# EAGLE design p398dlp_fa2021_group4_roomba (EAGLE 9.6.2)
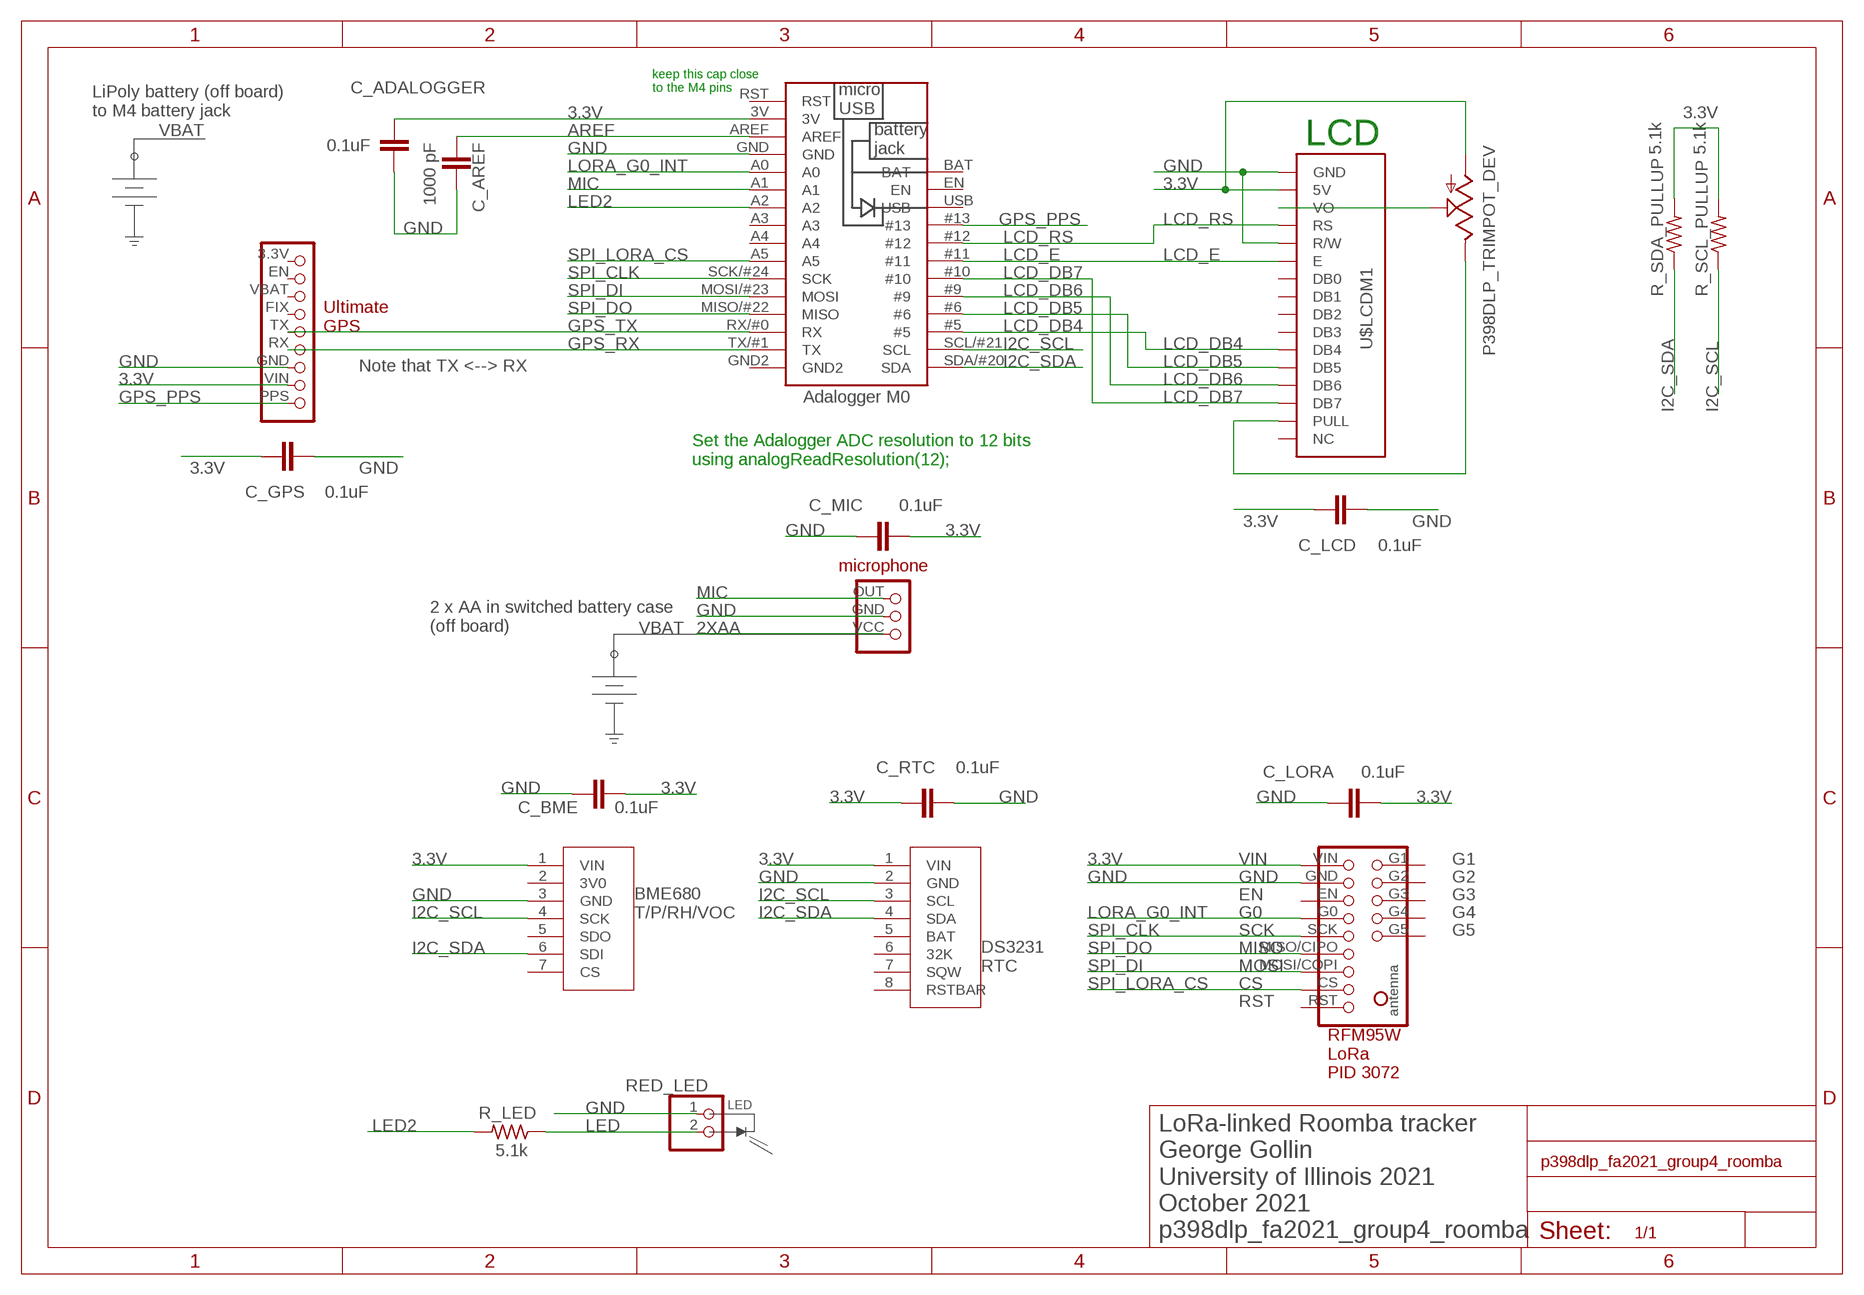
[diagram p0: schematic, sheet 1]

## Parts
BME  P398DLP_BME680_DEV  [P398DLP_BME680_PKG]
C_ADALOGGER  0.1uF  C5/3.5  [C5B3.5]
C_AREF  1000 pF  C5/3.5  [C5B3.5]
C_BME  0.1uF  C5/3.5  [C5B3.5]
C_GPS  0.1uF  C5/3.5  [C5B3.5]
C_LCD  0.1uF  C5/3.5  [C5B3.5]
C_LORA  0.1uF  C5/3.5  [C5B3.5]
C_MIC  0.1uF  C5/3.5  [C5B3.5]
C_RTC  0.1uF  C5/3.5  [C5B3.5]
DS3231  P398DLP_DS3231_DEV  [P398DLP_DS3231_PKG]
R_LED  5.1k  R-US_0207/7  [0207/7]
R_SCL_PULLUP  5.1k  R-US_0207/7  [0207/7]
R_SDA_PULLUP  5.1k  R-US_0207/7  [0207/7]
RED_LED  LED  PINHD-1X2  [1X02]
RFM95W  P398DLP_LORA_BREAKOUT_DEV  [P398DLP_LORA_BREAKOUT_PKG]
TRIMPOTADL1  P398DLP_TRIMPOT_DEV  [P398DLP_TRIMPOT_PKG]
U$2  P398DLP_ADALOGGER_MO_DEV  [P398DLP_ADALOGGER_M0_PKG]
U$7  P398DLP_MICROPHONE_DEV  [P398DLP_MICROPHONE_PKG]
U$16  P398DLP_ULTIMATE_GPS_DEV  [P398DLP_ULTIMATE_GPS_PKG]
U$LCDM1  P398DLP_LCD_16X2_DEV  [P398DLP_LCD_16X2_PKG]

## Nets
2XAA [power]: U$7.VCC
3.3V [power]: BME.1(VIN) C_ADALOGGER.1 C_BME.2 C_GPS.2 C_LCD.2 C_LORA.2 C_MIC.2 C_RTC.2 DS3231.1(VIN) R_SCL_PULLUP.2 R_SDA_PULLUP.2 RFM95W.VIN TRIMPOTADL1.BOTTOM U$2.3V U$16.VIN U$LCDM1.5V
AREF: C_AREF.1 U$2.AREF
GND [power]: BME.3(GND) C_ADALOGGER.2 C_AREF.2 C_BME.1 C_GPS.1 C_LCD.1 C_LORA.1 C_MIC.1 C_RTC.1 DS3231.2(GND) RED_LED.1 RFM95W.GND U$2.GND U$7.GND U$16.GND U$LCDM1.GND U$LCDM1.R/W
GPS_PPS: U$2.#13 U$16.PPS
GPS_RX: U$2.TX/#1(TX) U$16.RX
GPS_TX: U$2.RX/#0(RX) U$16.TX
I2C_SCL: BME.4(SCK) DS3231.3(SCL) R_SCL_PULLUP.1 U$2.SCL/#21(SCL)
I2C_SDA: BME.6(SDI) DS3231.4(SDA) R_SDA_PULLUP.1 U$2.SDA/#20(SDA)
LCD_DB4: U$2.#5 U$LCDM1.DB4
LCD_DB5: U$2.#6 U$LCDM1.DB5
LCD_DB6: U$2.#9 U$LCDM1.DB6
LCD_DB7: U$2.#10 U$LCDM1.DB7
LCD_E: U$2.#11 U$LCDM1.E
LCD_RS: U$2.#12 U$LCDM1.RS
LED2: R_LED.2 U$2.A2
LORA_G0_INT: RFM95W.G0 U$2.A0
MIC: U$2.A1 U$7.OUT
N$1: TRIMPOTADL1.TAP U$LCDM1.VO
N$4: TRIMPOTADL1.TOP U$LCDM1.PULL
N$34: R_LED.1 RED_LED.2
SPI_CLK: RFM95W.SCK U$2.SCK/#24(SCK)
SPI_DI: RFM95W.MOSI/COPI(MOSI) U$2.MOSI/#23(MOSI)
SPI_DO: RFM95W.MISO/CIPO(MISO) U$2.MISO/#22(MISO)
SPI_LORA_CS: RFM95W.CS U$2.A5
Unconnected: BME.2(3V0) BME.5(SDO) BME.7(CS) DS3231.5(BAT) DS3231.6(32K) DS3231.7(SQW) DS3231.8(RSTBAR) RFM95W.EN RFM95W.G1 RFM95W.G2 RFM95W.G3 RFM95W.G4 RFM95W.G5 RFM95W.RST U$2.A3 U$2.A4 U$2.BAT U$2.EN U$2.GND2 U$2.RST U$2.USB U$16.3.3V U$16.EN U$16.FIX U$16.VBAT U$LCDM1.DB0 U$LCDM1.DB1 U$LCDM1.DB2 U$LCDM1.DB3 U$LCDM1.NC

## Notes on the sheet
- keep this cap close 
  to the M4 pins
- LiPoly battery (off board)
  to M4 battery jack
- VBAT
- LCD
- Note that TX <--> RX
- Set the Adalogger ADC resolution to 12 bits 
  using analogReadResolution(12);
- 2 x AA in switched battery case
  (off board)
- VBAT
- LED
- LoRa-linked Roomba tracker
  George Gollin
  University of Illinois 2021
  October 2021
  p398dlp_fa2021_group4_roomba

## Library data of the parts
BME = p398dlp:P398DLP_BME680_DEV: BME680 temperature, pressure, relative humidity, and volatile organic compounds sensor
C_ADALOGGER C_AREF C_BME C_GPS C_LCD C_LORA C_MIC C_RTC = capacitor-wima:C: CAPACITOR
DS3231 = p398dlp:P398DLP_DS3231_DEV: DS3231 real time clock with battery backup
R_LED R_SCL_PULLUP R_SDA_PULLUP = resistor:R-US_: RESISTOR, American symbol
RED_LED = p398dlp:PINHD-1X2: PIN HEADER
RFM95W = p398dlp:P398DLP_LORA_BREAKOUT_DEV: LoRa 915 MHz breakout, Adafruit 3072
TRIMPOTADL1 = p398dlp_fa2019:P398DLP_TRIMPOT_DEV: trimpot
U$2 = p398dlp:P398DLP_ADALOGGER_MO_DEV: Adafruit Adalogger M0 processor
U$7 = p398dlp:P398DLP_MICROPHONE_DEV: Adafruit amplified electret microphone
U$16 = p398dlp:P398DLP_ULTIMATE_GPS_DEV: Adafruit "ultimate GPS" breakout board
U$LCDM1 = p398dlp:P398DLP_LCD_16X2_DEV: 2x16 liquid crystal display, four mounting holes

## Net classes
1 power: width 0.305 mm

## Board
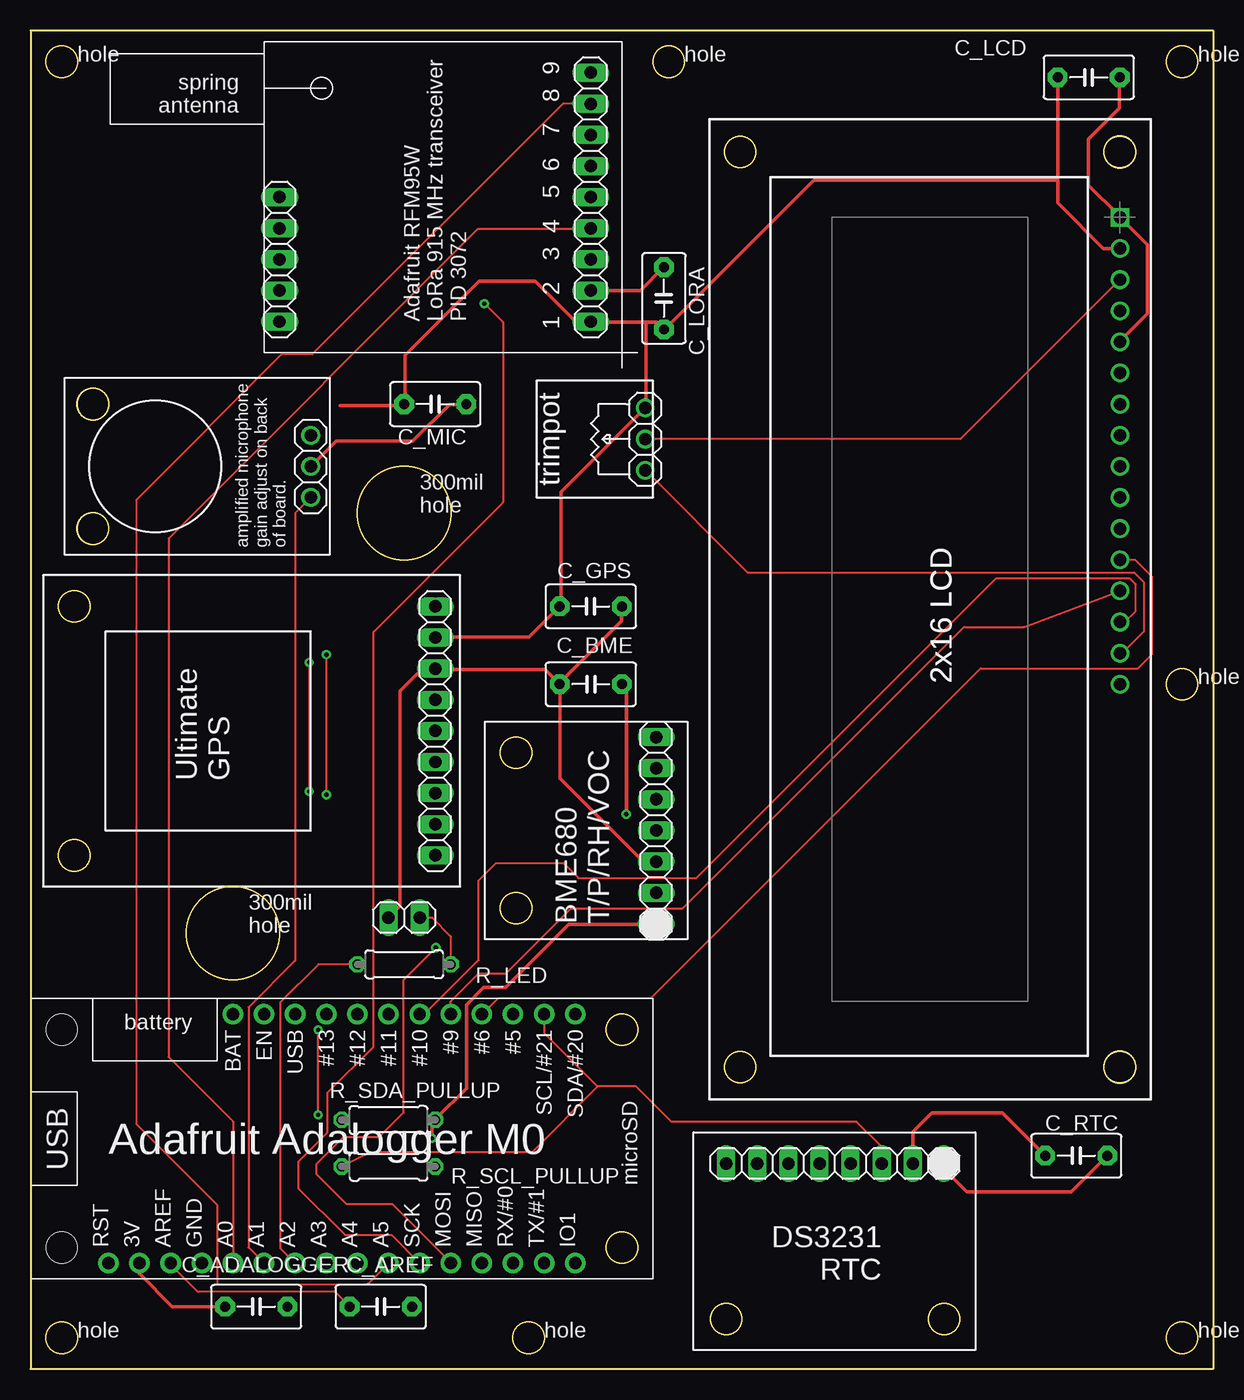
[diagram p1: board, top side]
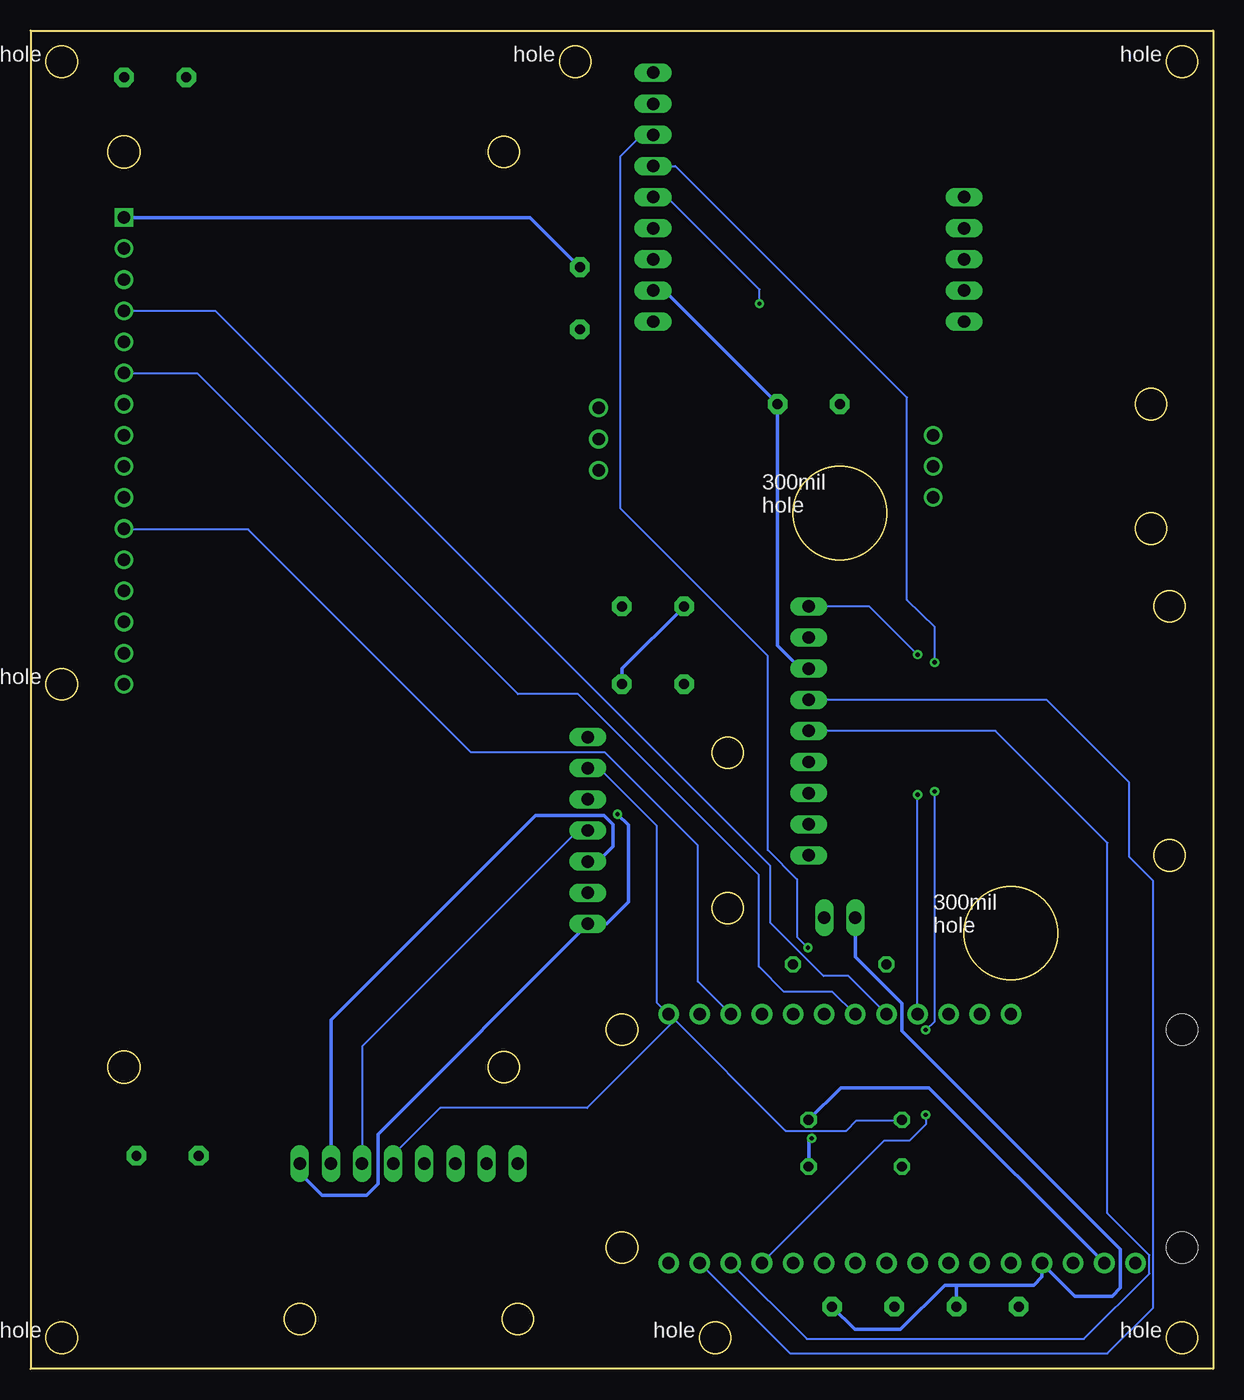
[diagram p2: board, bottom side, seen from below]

Size 96.52 x 109.22 mm. Coordinates in mm from the lower left corner, seen from the top.
Outline: 0,0 96.52,0 96.52,109.22 0,109.22 0,0
Copper layers (1*16): Top 0.035mm / dielectric 0.2mm / Bottom 0.035mm
Design rules "default *": minimum track width 6mil, minimum drill 0.35mm, track to track 6mil, track to pad 6mil, pad to pad 6mil, via to via 6mil, smd to smd 6mil, copper to edge 40mil, drill to drill 6mil, minimum pad ring 10mil, minimum via ring 8mil, stop-mask expansion 4mil, vias tented up to drill 0mil, thermal gap 10mil

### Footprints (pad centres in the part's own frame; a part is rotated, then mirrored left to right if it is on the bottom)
P398DLP_BME680_PKG = drill 1.016 long: 1 0,0; 2 2.54,0; 3 5.08,0; 4 7.62,0; 5 10.16,0; 6 12.7,0; 7 15.24,0 | hole 2.54: 1.27,11.43; 13.97,11.43
C5B3.5 = drill 0.813 pad 1.6 octagon: 1 -2.54,0; 2 2.54,0
P398DLP_DS3231_PKG = drill 1.016 long: 1 0,0; 2 2.54,0; 3 5.08,0; 4 7.62,0; 5 10.16,0; 6 12.7,0; 7 15.24,0; 8 17.78,0 | hole 2.54: 0,12.7; 17.78,12.7
0207/7 = drill 0.813 octagon: 1 -3.81,0; 2 3.81,0
1X02 = drill 1.016 long: 1 -1.27,0; 2 1.27,0
P398DLP_LORA_BREAKOUT_PKG = drill 1.016 long: CS 20.32,2.54; EN 7.62,2.54; G0 10.16,2.54; G1 2.54,27.94; G2 5.08,27.94; G3 7.62,27.94; G4 10.16,27.94; G5 12.7,27.94; GND 5.08,2.54; MISO/CIPO 15.24,2.54; MOSI/COPI 17.78,2.54; RST 22.86,2.54; SCK 12.7,2.54; VIN 2.54,2.54
P398DLP_TRIMPOT_PKG = drill 1.016: BOTTOM 7.303,0.635; TAP 4.763,0.635; TOP 2.223,0.635
P398DLP_ADALOGGER_M0_PKG = drill 1 pad 1.676: 3V 8.89,1.27; #5 39.37,21.59; #6 36.83,21.59; #9 34.29,21.59; #10 31.75,21.59; #11 29.21,21.59; #12 26.67,21.59; #13 24.13,21.59; A0 16.51,1.27; A1 19.05,1.27; A2 21.59,1.27; A3 24.13,1.27; A4 26.67,1.27; A5 29.21,1.27; AREF 11.43,1.27; BAT 16.51,21.59; EN 19.05,21.59; GND 13.97,1.27; GND2 44.45,1.27; MISO/#22 36.83,1.27; MOSI/#23 34.29,1.27; RST 6.35,1.27; RX/#0 39.37,1.27; SCK/#24 31.75,1.27; SCL/#21 41.91,21.59; SDA/#20 44.45,21.59; TX/#1 41.91,1.27; USB 21.59,21.59 | hole 2.54: 48.26,2.54; 48.26,20.32; 2.54,20.32; 2.54,2.54
P398DLP_MOUNTING_HOLE_PKG = hole 2.54: 0,0
P398DLP_MOUNTING_HOLE_300MIL_PKG = hole 7.62: 0,0
P398DLP_MICROPHONE_PKG = drill 1.016: GND 2.54,0; OUT 0,0; VCC 5.08,0 | hole 2.54: -2.54,17.78; 7.62,17.78
P398DLP_ULTIMATE_GPS_PKG = drill 1.016 long: 3.3V 0,0; EN 2.54,0; FIX 7.62,0; GND 15.24,0; PPS 20.32,0; RX 12.7,0; TX 10.16,0; VBAT 5.08,0; VIN 17.78,0 | hole 2.54: 0,29.464; 20.32,29.464
P398DLP_LCD_16X2_PKG = drill 1.016: 5V 2.544,0.006; DB0 15.244,0.006; DB1 17.784,0.006; DB2 20.324,0.006; DB3 22.864,0.006; DB4 25.404,0.006; DB5 27.944,0.006; DB6 30.484,0.006; DB7 33.024,0.006; E 12.704,0.006; NC 38.104,0.006; PULL 35.564,0.006; R/W 10.164,0.006; RS 7.624,0.006; VO 5.084,0.006 | drill 1.016 square: GND 0.004,0.006 | hole 2.54: -5.334,0; -5.334,-30.988; 69.342,-30.988; 69.342,0

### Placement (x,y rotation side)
BME  51.05,36.32 90 top
C_ADALOGGER  18.41,5.08 0 top
C_AREF  28.57,5.08 0 top
C_BME  45.72,55.88 0 top
C_GPS  45.72,62.23 180 top
C_LCD  86.36,105.41 180 top
C_LORA  51.69,87.38 270 top
C_MIC  33.02,78.74 180 top
C_RTC  85.34,17.4 0 top
DS3231  74.55,16.76 180 top
R_LED  30.48,33.02 180 top
R_SCL_PULLUP  29.21,16.51 0 top
R_SDA_PULLUP  29.21,20.32 0 top
RED_LED  30.48,36.83 0 top
RFM95W  48.26,82.93 90 top
TRIMPOTADL1  50.8,71.12 90 top
U$2  0,7.37 0 top
U$3  [P398DLP_MOUNTING_HOLE_PKG]  93.98,2.54 0 top
U$4  [P398DLP_MOUNTING_HOLE_PKG]  2.54,2.54 0 top
U$5  [P398DLP_MOUNTING_HOLE_PKG]  40.64,2.54 0 top
U$6  [P398DLP_MOUNTING_HOLE_300MIL_PKG]  16.51,35.56 0 top
U$7  22.86,71.12 90 top
U$11  [P398DLP_MOUNTING_HOLE_PKG]  93.98,106.68 0 top
U$12  [P398DLP_MOUNTING_HOLE_PKG]  52.07,106.68 0 top
U$13  [P398DLP_MOUNTING_HOLE_PKG]  93.98,55.88 0 top
U$16  33.02,41.91 90 top
U$22  [P398DLP_MOUNTING_HOLE_PKG]  2.54,106.68 0 top
U$24  [P398DLP_MOUNTING_HOLE_300MIL_PKG]  30.48,69.85 0 top
U$LCDM1  88.9,93.98 270 top

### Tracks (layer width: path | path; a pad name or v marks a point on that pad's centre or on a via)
3.3V  (via drill 0.35)
  Top 0.305: DS3231.1 74.55,16.31 76.4,14.45 84.94,14.45 C_RTC.2 | 11.56,5.08 8.89,7.75 U$2.3V | C_ADALOGGER.1 11.56,5.08 | 11.56,5.08 | v32.77,18.82 32.77,20.04 32.99,20.27 R_SDA_PULLUP.2 33.07,20.42 35.56,22.91 35.56,29.69 36.98,31.11 38.76,31.11 43.92,36.27 51.05,36.27 BME.1 | U$16.VIN 33.07,59.74 40.69,59.74 C_GPS.2 43.28,62.33 43.28,71.55 50.06,78.33 TRIMPOTADL1.BOTTOM 50.22,78.49 50.22,85.42 | U$LCDM1.5V 87.56,91.44 83.82,95.17 83.82,97.08 | C_LCD.2 83.82,97.08 | 25.27,78.61 30.38,78.61 30.48,78.72 C_MIC.2 30.56,78.87 30.56,82.73 36.6,88.77 41.17,88.77 44.48,85.47 RFM95W.VIN 45.72,85.42 50.22,85.42 | 50.22,85.42 51.13,85.42 51.66,84.89 C_LORA.2 51.82,84.89 63.93,97 83.74,97 83.82,97.08 | v48.62,45.26 48.62,55.55 48.31,55.85 C_BME.2
  Bottom 0.305: v32.77,18.82 32.99,18.59 32.99,16.54 R_SCL_PULLUP.2 | R_SDA_PULLUP.2 30.4,22.94 23.19,22.94 8.94,8.69 8.91,8.69 U$2.3V | DS3231.1 74.55,16 72.72,14.17 69.09,14.17 68.17,15.09 68.17,19.15 51.05,36.27 BME.1 49.53,36.32 47.73,38.12 47.73,44.37 v48.62,45.26 | C_BME.2 48.23,55.93 48.23,57.15 43.2,62.18 C_GPS.2
AREF
  Top 0.152: C_AREF.1 24.84,6.27 13.64,6.27 11.43,8.48 U$2.AREF
GND
  Top 0.305: U$LCDM1.R/W 88.92,83.82 88.92,83.92 91.14,86.13 91.14,91.75 88.92,93.95 U$LCDM1.GND 88.85,94.11 86.33,96.62 86.33,100.36 88.85,102.87 88.85,105.39 C_LCD.1 | RFM95W.GND 49.76,88.01 51.66,89.92 C_LORA.1 | U$7.GND 24.92,75.72 31.19,75.72 34.19,78.72 35.51,78.72 C_MIC.1 | RED_LED.1 30.15,37.77 30.15,55.32 31.98,57.15 U$16.GND 33.15,57.07 41.99,57.07 C_BME.1 | DS3231.2 72.01,19.33 73.56,20.88 79.32,20.88 C_RTC.1 | BME.3 49.99,41.4 43.2,48.18 43.2,55.85 C_BME.1 | C_GPS.1 48.23,62.18 48.23,61.04 43.2,56.01 C_BME.1
  Bottom 0.305: RFM95W.GND 44.81,88.01 35.59,78.79 C_MIC.1 35.59,78.64 35.59,59.03 33.71,57.15 U$16.GND | U$LCDM1.GND 88.85,93.95 55.78,93.95 51.74,89.92 C_LORA.1 | 20.95,6.83 C_ADALOGGER.2 | 20.95,6.83 14.66,6.83 13.97,7.52 U$2.GND 11.28,5.94 8.26,5.94 7.57,6.63 7.57,9.75 25.4,27.58 25.4,29.84 29.18,33.63 29.18,36.8 RED_LED.1 | 20.95,6.83 21.92,6.83 25.53,3.23 29.26,3.23 C_AREF.2 | DS3231.2 72.01,28.47 55.32,45.16 49.71,45.16 48.97,44.42 48.97,42.65 50.22,41.4 BME.3
GPS_PPS  (via drill 0.35)
  Top 0.152: v24.13,58.29 v24.13,46.86
  Bottom 0.152: U$2.#13 v24.13,46.86 | v24.13,58.29 28.07,62.23 U$16.PPS
GPS_RX
  Bottom 0.152: U$2.TX/#1 34.54,1.27 8.64,1.27 4.9,5 4.9,39.83 6.86,41.78 6.86,47.88 13.59,54.61 U$16.RX
GPS_TX
  Bottom 0.152: U$2.RX/#0 33.17,2.44 10.54,2.44 5.21,7.77 5.21,9.27 8.64,12.7 8.64,42.93 17.78,52.07 U$16.TX
I2C_SCL
  Top 0.152: 46.28,23.04 40.92,17.68 27.74,17.68 R_SCL_PULLUP.1 | U$2.SCL/#21 41.91,27.41 46.28,23.04 | 46.28,23.04 49.43,23.04 52.3,20.17 67.41,20.17 69.47,18.11 DS3231.3
  Bottom 0.152: BME.4 51.28,43.71 52.07,43.71 69.42,26.36 69.42,16.76 DS3231.3
I2C_SDA
  Bottom 0.152: R_SDA_PULLUP.1 25.45,20.27 29.11,20.27 29.95,19.43 34.9,19.43 44.42,28.96 U$2.SDA/#20 | DS3231.4 66.93,17.45 63.09,21.29 51.1,21.29 43.97,28.42 U$2.SDA/#20 | BME.6 50.11,49.02 45.41,44.32 45.41,29.87 44.5,28.96 U$2.SDA/#20
LCD_DB4
  Bottom 0.152: U$LCDM1.DB4 88.85,68.5 78.77,68.5 60.58,50.32 49.66,50.32 42.06,42.72 42.06,31.62 39.4,28.96 U$2.#5
LCD_DB5
  Top 0.152: U$LCDM1.DB5 90.12,66.04 91.54,64.62 91.54,58.34 90.37,57.17 77.52,57.17 50.62,30.28 38.2,30.28 36.88,28.96 U$2.#6
LCD_DB6
  Top 0.152: U$2.#9 34.29,29.97 36.58,32.26 38.79,32.26 44.12,37.59 53.21,37.59 76.17,60.55 81.1,60.55 U$LCDM1.DB6
LCD_DB7
  Top 0.152: U$LCDM1.DB7 89.3,60.96 90.17,61.82 90.17,64.06 89.69,64.54 78.82,64.54 54.33,40.06 44.7,40.06 43.48,41.27 37.97,41.27 36.58,39.88 36.58,33.38 32.16,28.96 U$2.#10
LCD_E
  Bottom 0.152: U$LCDM1.E 88.85,81.23 82.91,81.23 56.74,55.07 51.84,55.07 37.08,40.31 37.08,32.84 35.03,30.79 31.09,30.79 29.26,28.96 U$2.#11
LCD_RS
  Bottom 0.152: U$2.#12 29.77,32.05 31.8,32.05 36.14,36.4 36.14,41.05 81.43,86.33 88.85,86.33 U$LCDM1.RS
LED2
  Top 0.152: R_LED.2 23.5,33.02 20.37,29.9 20.37,9.86 U$2.A2
LORA_G0_INT
  Top 0.152: U$2.A0 16.51,20.19 11.25,25.45 11.25,67.77 36.52,93.04 45.72,93.04 RFM95W.G0
MIC
  Top 0.152: U$7.OUT 21.59,69.85 21.59,33.33 17.78,29.52 17.78,9.91 U$2.A1
N$1
  Top 0.152: TRIMPOTADL1.TAP 50.22,75.89 75.89,75.89 88.85,88.85 U$LCDM1.VO
N$4
  Top 0.152: U$LCDM1.PULL 89.1,58.42 90.86,60.17 90.86,64.21 90.07,65 58.52,65 50.22,73.3 TRIMPOTADL1.TOP
N$34
  Top 0.152: R_LED.1 34.29,35.31 32.77,36.83 RED_LED.2
SPI_CLK  (via drill 0.35)
  Top 0.152: v37.03,86.94 38.56,85.42 38.56,70.71 27.99,60.15 27.99,26.29 24.22,22.52 24.22,19.27 21.84,16.89 21.84,14.73 25.65,10.92 29.46,10.92 U$2.SCK/#24
  Bottom 0.152: RFM95W.SCK 44.58,95.63 37.03,88.09 v37.03,86.94
SPI_DI  (via drill 0.35)
  Top 0.152: v33.07,34.37 30.45,31.75 30.45,20.93 28.45,18.92 25.53,18.92 23.36,16.75 23.36,15.86 25.78,13.44 29.54,13.44 34.29,8.69 U$2.MOSI/#23
  Bottom 0.152: RFM95W.MOSI/COPI 46.63,100.71 48.36,98.98 48.36,70.21 36.35,58.19 36.35,42.34 33.96,39.95 33.96,35.26 v33.07,34.37
SPI_DO  (via drill 0.35)
  Top 0.152: v23.47,20.73 v23.47,27.66 | v22.73,57.66 v22.73,47.12
  Bottom 0.152: RFM95W.MISO/CIPO 43.89,98.17 24.99,79.27 24.99,62.76 22.73,60.53 v22.73,57.66 | v22.73,47.12 22.73,28.37 v23.47,27.66 | v23.47,20.73 23.47,19.94 24.77,18.64 26.85,18.64 36.8,8.69 U$2.MISO/#22
SPI_LORA_CS
  Top 0.152: RFM95W.CS 43.43,103.25 22.99,82.8 20.5,82.8 8.66,70.97 8.66,19.94 15.2,13.4 15.2,6.91 27.48,6.91 U$2.A5

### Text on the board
tDocu: p398dlp_fa2021_group4_roomba | George Gollin / University of Illinois / Fille de Lear Designs / October 2021 | JLCJLCJLCJLC | longer / leg
bDocu: p398dlp_fa2021_group4_roomba | George Gollin / University of Illinois / Fille de Lear Designs / October 2021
